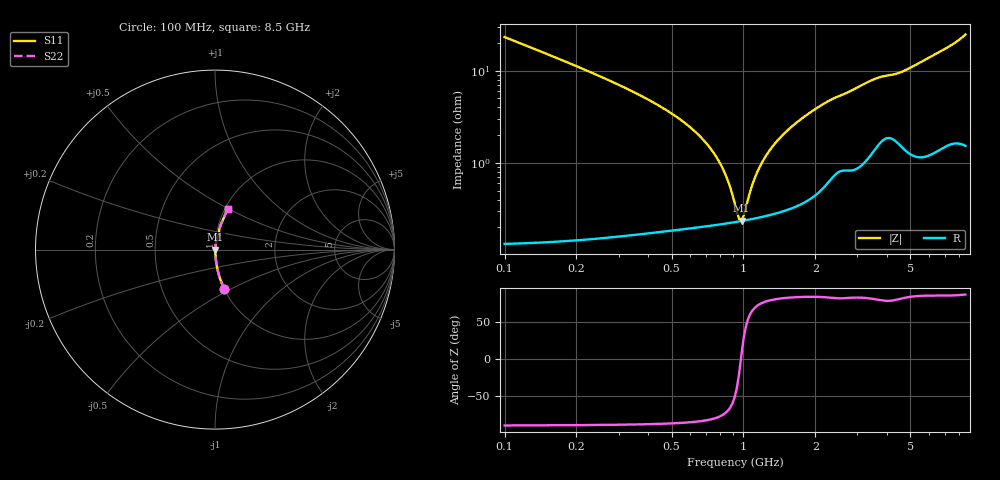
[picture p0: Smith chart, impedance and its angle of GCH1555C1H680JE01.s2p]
!Murata Part Number: GCH1555C1H680JE01
!These Parameters are Measured in Series Mode Connection
!Data Generated on Jun 19, 2026
!  o--ll--o
!Port1  Port2
!  o------o
!Operation Temp=25[degC], DC Bias Voltage=0[V]
!Freq. Start=100[MHz] Stop=9[GHz] 401[Steps]
# Hz S RI R 50
!Freq.(Hz) S11(Real) S11(Imag) S21(Real) S21(Imag) S12(Real) S12(Imag) S22(Real) S22(Imag)
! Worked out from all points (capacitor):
!   401 points, 100 MHz to 8.5 GHz, reference 50 ohm
!   read as one part in series: C = 68.1 pF near 142 MHz
!   lowest |Z| = 237 mohm at 982 MHz (marker M1)
!   series resonance near 976.5 MHz, so ESL is about 390 pH
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1e8  0.052 -0.2191  0.948 0.2191  0.948 0.2191  0.052 -0.2191
2.05e8  0.0131 -0.1073  0.9869 0.1073  0.9869 0.1073  0.0131 -0.1073
2.89e8  0.00694 -0.073  0.9931 0.073  0.9931 0.073  0.00694 -0.073
6.04e8  0.00252 -0.0237  0.9975 0.0237  0.9975 0.0237  0.00252 -0.0237
7.3e8  0.00228 -0.014  0.9977 0.014  0.9977 0.014  0.00228 -0.014
8.35e8  0.00225 -0.00746  0.9978 0.00746  0.9978 0.00746  0.00225 -0.00746
9.4e8  0.0023 -0.00181  0.9977 0.00181  0.9977 0.00181  0.0023 -0.00181
9.61e8  0.00232 -0.000756  0.9977 0.000756  0.9977 0.000756  0.00232 -0.000756
9.82e8  0.00234 0.000271  0.9977 -0.000271  0.9977 -0.000271  0.00234 0.000271
1.024e9  0.0024 0.00226  0.9976 -0.00226  0.9976 -0.00226  0.0024 0.00226
1.108e9  0.00252 0.00603  0.9975 -0.00603  0.9975 -0.00603  0.00252 0.00603
1.192e9  0.00268 0.00956  0.9973 -0.00956  0.9973 -0.00956  0.00268 0.00956
1.318e9  0.00297 0.0145  0.997 -0.0145  0.997 -0.0145  0.00297 0.0145
1.507e9  0.00351 0.0214  0.9965 -0.0214  0.9965 -0.0214  0.00351 0.0214
1.78e9  0.0046 0.0307  0.9954 -0.0307  0.9954 -0.0307  0.0046 0.0307
2.116e9  0.00676 0.0413  0.9932 -0.0413  0.9932 -0.0413  0.00676 0.0413
2.914e9  0.0122 0.0614  0.9878 -0.0614  0.9878 -0.0614  0.0122 0.0614
3.586e9  0.0205 0.0783  0.9795 -0.0783  0.9795 -0.0783  0.0205 0.0783
4.3e9  0.0248 0.0862  0.9752 -0.0862  0.9752 -0.0862  0.0248 0.0862
5.707e9  0.0273 0.124  0.9727 -0.124  0.9727 -0.124  0.0273 0.124
7.114e9  0.044 0.1664  0.956 -0.1664  0.956 -0.1664  0.044 0.1664
8.5e9  0.0699 0.2257  0.9301 -0.2257  0.9301 -0.2257  0.0699 0.2257
